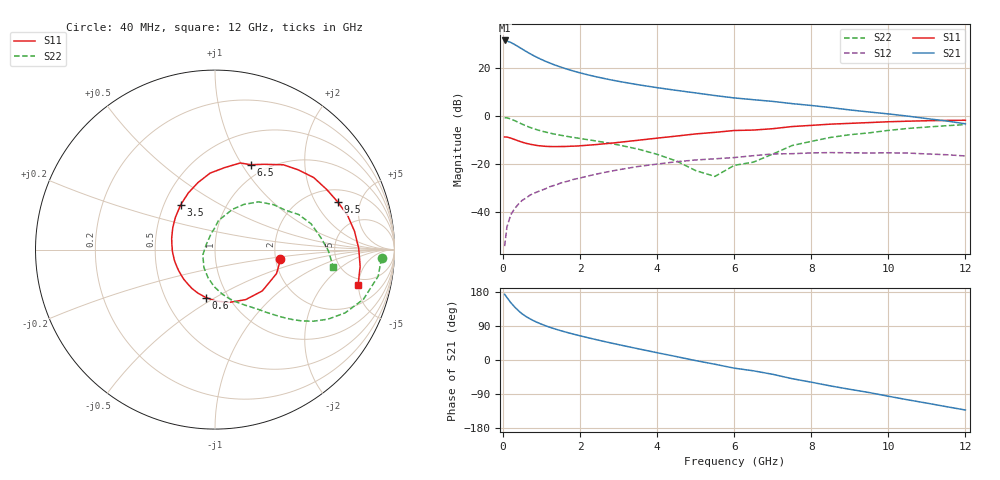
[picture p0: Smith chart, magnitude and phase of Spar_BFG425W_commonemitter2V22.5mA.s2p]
! Filename: 222bfg425.001
! BFG425W Field C1
! V1=8.645E-001V,V2=2.000E+000V, I1=3.197E-004A, I2=2.246E-002A
# GHz  S  MA  R 50
!  S11  S21  S12  S22
!Freq(GHz)  Mag  Ang  Mag  Ang  Mag  Ang  Mag  Ang
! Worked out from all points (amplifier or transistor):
!   44 points, 40 MHz to 12 GHz, reference 50 ohm
!   highest |S21| = 31.4 dB at 40 MHz (marker M1)
!   |S21| within 3 dB of that: start of sweep to 438 MHz
!   unconditionally stable (mu >= 1): 1.236 GHz to end of sweep
!   at 700 MHz: K = 0.78, MSG = 29.3 dB, |S12| = -32.8 dB
!   at 2.4 GHz: K = 1.16, MAG = 17.8 dB, |S12| = -24.2 dB
!   at 12 GHz: K = 1.34, MAG = 3.2 dB, |S12| = -16.5 dB
!   S11 on the Smith chart (normalised r, x): 40 MHz: 2.13, -0.27; 600 MHz: 0.79, -0.46; 3.5 GHz: 0.61, +0.34; 6.5 GHz: 0.85, +1.09; 9.5 GHz: 2.73, +3.12; 12 GHz: 4.14, -4.94
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0.04  0.369 -8.6  37.13 173.5  0.002 83.6  0.929 -3.0
0.1  0.368 -21.3  36.14 165.0  0.005 83.5  0.921 -9.3
0.2  0.35 -41.1  33.72 151.4  0.009 75.9  0.872 -18.5
0.3  0.327 -58.4  30.61 139.9  0.012 71.3  0.806 -26.0
0.4  0.305 -74.4  27.43 130.0  0.015 68.0  0.739 -31.7
0.5  0.287 -88.8  24.51 121.4  0.018 65.4  0.678 -36.0
0.6  0.272 -100.6  21.93 114.5  0.02 63.7  0.626 -39.4
0.7  0.261 -111.0  19.73 108.6  0.023 62.4  0.582 -42.1
0.8  0.252 -120.6  17.86 103.2  0.025 61.6  0.546 -44.2
0.9  0.244 -128.8  16.28 98.6  0.027 60.8  0.515 -46.2
1.2  0.234 -149.2  12.74 86.9  0.034 58.7  0.447 -51.1
1.6  0.234 -170.3  9.778 74.4  0.043 55.9  0.387 -56.8
2.2  0.249 165.8  7.189 58.9  0.057 50.0  0.324 -66.1
2.8  0.274 146.3  5.647 44.9  0.072 42.8  0.27 -76.7
3.5  0.315 127.3  4.487 29.7  0.09 33.2  0.207 -91.1
4.5  0.385 104.3  3.421 8.9  0.113 18.1  0.117 -122.0
5.5  0.46 83.3  2.67 -11.2  0.13 2.3  0.056 151.1
6.5  0.513 67.2  2.189 -28.6  0.151 -10.3  0.111 93.6
8.5  0.681 36.1  1.503 -68.4  0.175 -47.1  0.361 47.5
9.5  0.734 21.1  1.217 -85.8  0.172 -63.6  0.449 29.3
10.5  0.784 7.5  1.001 -105.0  0.171 -82.0  0.554 15.1
12  0.821 -13.7  0.692 -132.0  0.149 -111.3  0.667 -8.5
